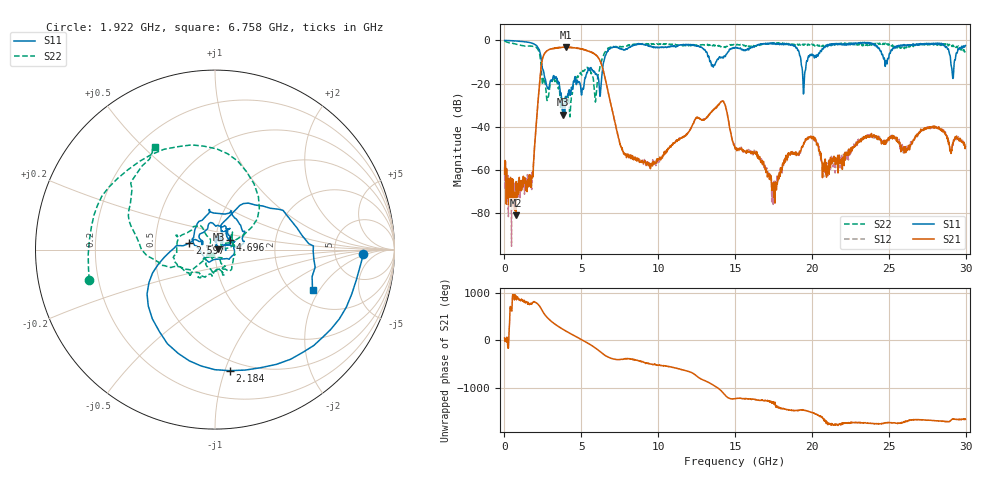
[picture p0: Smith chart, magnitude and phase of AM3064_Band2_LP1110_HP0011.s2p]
# Hz S DB R 50.0
!freq dBS11 angS11 dBS21 angS21 dBS12 angS12 dBS22 angS22
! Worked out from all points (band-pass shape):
!   1600 points, 10 MHz to 29.98 GHz, reference 50 ohm
!   highest |S21| = -3.11 dB at 4.002 GHz (marker M1); lowest = -81.2 dB at 741 MHz (marker M2)
!   |S21| within 3 dB of the highest: 2.608 GHz to 5.83 GHz (3.222 GHz wide, 76.4 % of centre)
!   lowest |S11| = -34.4 dB at 3.815 GHz (marker M3), VSWR 1.04, Z = 51.9 + j0.111 ohm
!   |S11| at or under -10 dB: 2.414 GHz to 6.455 GHz (4.041 GHz wide, 91.1 % of centre); 13.42 GHz to 13.77 GHz (340.7 MHz wide, 2.51 % of centre); 19.29 GHz to 19.64 GHz (349.7 MHz wide, 1.8 % of centre)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
!   |S22| runs from -35.5 to -0.3 dB; largest |S21 - S12| = 0.023
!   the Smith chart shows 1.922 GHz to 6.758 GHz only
!   S11 on the Smith chart (normalised r, x): 1.922 GHz: 10, -2; 2.184 GHz: 0.41, -1.04; 2.597 GHz: 0.75, +0.05; 4.696 GHz: 1.17, +0.13; 6.758 GHz: 2.54, -1.73
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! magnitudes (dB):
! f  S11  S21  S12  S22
! 10 MHz  0.0  -62.1  -58.6  -0.3
! 741 MHz  -0.3  -81.2  -68.8  -1.7
! 1.922 GHz  -1.6  -53.4  -53.7  -2.8
! 2.184 GHz  -3.4  -28.2  -28.2  -4.3
! 2.597 GHz  -16.6  -6.2  -6.2  -18.8
! 3.815 GHz  -34.4  -3.2  -3.2  -30.5
! 4.002 GHz  -26.3  -3.1  -3.2  -27.3
! 4.696 GHz  -20.2  -3.5  -3.6  -18.0
! 5.015 GHz  -25.4  -4.1  -3.9  -16.0
! 5.933 GHz  -15.8  -6.6  -6.6  -28.0
! 6.758 GHz  -4.6  -24.4  -24.4  -3.6
! 7.789 GHz  -4.3  -52.2  -52.6  -2.8
! 10 GHz  -3.4  -55.1  -54.8  -1.8
! 14.14 GHz  -7.8  -28.2  -28.3  -3.0
! 15 GHz  -3.3  -49.7  -49.5  -1.9
! 17.54 GHz  -1.6  -72.9  -65.3  -1.2
! 19.47 GHz  -24.1  -47.5  -47.9  -2.3
! 19.99 GHz  -6.4  -44.9  -44.9  -1.7
! 20.89 GHz  -2.5  -60.3  -60.3  -2.9
! 25 GHz  -8.0  -45.7  -45.5  -1.6
! 29.18 GHz  -17.7  -48.0  -48.5  -2.2
! 29.98 GHz  -2.4  -49.4  -49.3  -4.5
